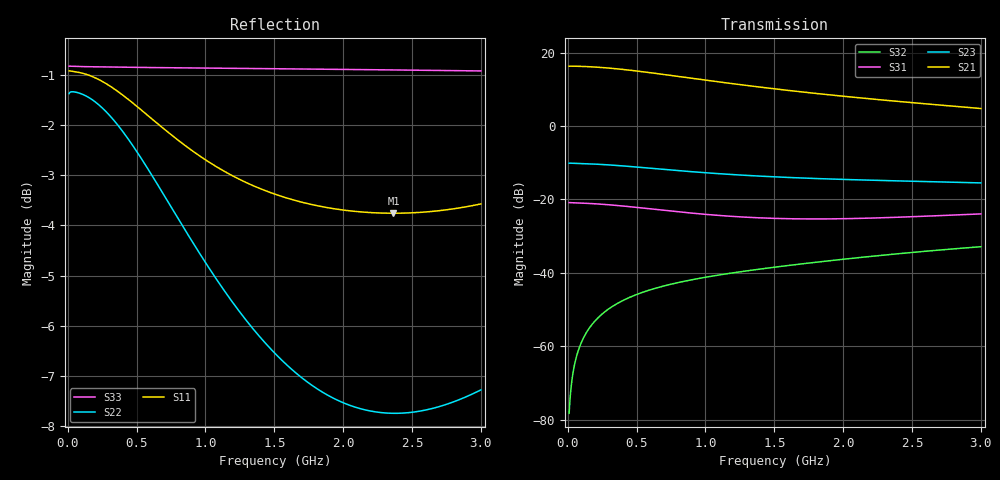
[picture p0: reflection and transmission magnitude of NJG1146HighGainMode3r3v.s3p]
! Created Mon Oct 18 18:43:47 2010
# hz S ma R 50
! 3 Port Network Data Port1:RFIN  Port2:RFOUT1  Port3:RFOUT2
! freq  magS11  angS11  magS12  angS12  magS13  angS13
!  magS21  angS21
!  magS22  angS22  magS23  angS23
!  magS31  angS31  magS32  angS32
!  magS33  angS33
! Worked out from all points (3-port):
!   2991 points, 10 MHz to 3 GHz, reference 50 ohm
!   strongest paths, dB at 10 MHz, 757 MHz, 1.505 GHz, 2.253 GHz, 3 GHz:
!     S21: 16.3, 13.7, 10.1, 7.2, 4.8
!     S23: -10.1, -12.0, -13.9, -14.8, -15.5
!     S31: -20.9, -23.2, -25.2, -25.0, -24.0
!     S32: -78.3, -43.1, -38.5, -35.3, -32.9
!   lowest |S11| = -3.8 dB at 2.365 GHz (marker M1), VSWR 4.69, Z = 11.6 - j14.7 ohm
!   |S11| at or under -10 dB: nowhere
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1e7  0.8994 -1.2  0.00193 57.5  0.09036 -0.4
     6.514 179.5  0.8536 -0.1  0.3111 179.7
     0.09035 -0.5  0.0001216 64.7  0.9091 -0.1
4.6e7  0.8979 -5.5  0.007643 79.3  0.0897 -1.6
       6.523 176.0  0.857 -2.6  0.3098 177.2
       0.0897 -2.0  0.0005219 83.0  0.9085 -0.4
9.8e7  0.8951 -11.5  0.01612 79.9  0.08908 -2.8
       6.486 171.3  0.8533 -5.9  0.3075 174.3
       0.08896 -3.7  0.001113 83.4  0.9082 -0.8
3.13e8  0.8674 -35.7  0.04898 68.4  0.08553 -7.6
        6.118 152.8  0.8094 -18.2  0.2936 163.0
        0.08398 -10.1  0.003368 77.5  0.9073 -2.5
5.88e8  0.8105 -62.7  0.08181 53.7  0.0786 -11.4
        5.355 132.2  0.7161 -30.9  0.267 151.1
        0.07473 -15.0  0.005771 72.1  0.9063 -4.6
7.79e8  0.7713 -78.3  0.09828 45.3  0.07398 -12.3
        4.798 120.1  0.6485 -37.4  0.2486 144.6
        0.06847 -16.0  0.007192 69.8  0.9057 -6.0
1.02e9  0.7303 -94.6  0.1136 36.7  0.06937 -12.0
        4.166 107.0  0.5738 -43.3  0.2292 137.9
        0.06204 -15.1  0.008817 68.1  0.905 -7.9
1.505e9  0.6777 -119.0  0.1342 23.8  0.06429 -9.1
         3.201 85.5  0.4703 -49.7  0.2026 127.1
         0.05507 -9.1  0.01193 66.3  0.9038 -11.5
2.365e9  0.6487 -145.6  0.1574 6.3  0.06422 -4.6
         2.19 54.8  0.41 -53.7  0.1792 109.2
         0.05681 1.5  0.01791 62.5  0.9013 -18.1
3e9  0.6628 -158.3  0.169 -6.5  0.06752 -4.7
     1.729 33.8  0.4326 -58.1  0.1676 94.4
     0.06338 3.0  0.02264 56.7  0.8992 -22.9
